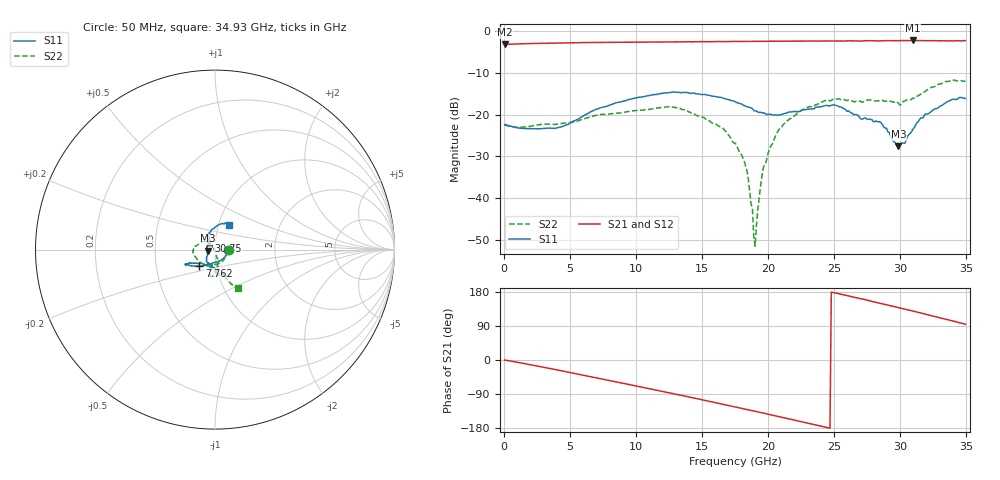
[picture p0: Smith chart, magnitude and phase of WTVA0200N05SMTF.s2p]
! 50 ohm 2-Port S-parameters measured by Modelithics Inc support@modelithics.com  Tampa, FL USA 813-866-6335 (February 2024)
! Smiths Interconnect,  2dB P/N: WTVA0200N05SMTF, Temperature: -50 C
! Board: 10 mil Rogers 4350B, Mounting Pad Dimensions: Length: 15 mils, Width: 25 mils, Gap: 40 mils.
# Hz S RI R 50
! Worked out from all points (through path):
!   352 points, 50 MHz to 34.93 GHz, reference 50 ohm
!   highest |S21| = -2.32 dB at 30.95 GHz (marker M1); lowest = -3.3 dB at 50 MHz (marker M2)
!   group delay of S21, straight-line fit = 21.1 ps
!   lowest |S11| = -27.6 dB at 29.85 GHz (marker M3), VSWR 1.09, Z = 46 - j0.582 ohm
!   |S11| at or under -10 dB: start of sweep to end of sweep
!   |S22| runs from -51.4 to -11.8 dB; largest |S21 - S12| = 0.0048
!   S11 on the Smith chart (normalised r, x): 50 MHz: 1.16, -0.01; 7.762 GHz: 0.83, -0.15; 30.75 GHz: 0.93, +0.09; 34.93 GHz: 1.12, +0.31
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5e7  0.0752 -0.00255  0.686 -0.00206  0.6856 -0.00233  0.0757 -0.00234
3.8815e9  0.0104 -0.0676  0.6451 -0.3032  0.6446 -0.3035  0.0314 -0.0696
5.8715e9  -0.0415 -0.0838  0.56 -0.4554  0.5597 -0.4554  -0.0087 -0.0868
7.762e9  -0.0866 -0.091  0.4415 -0.577  0.4415 -0.5768  -0.048 -0.0888
1.1742e10  -0.1548 -0.0845  0.1121 -0.7237  0.1112 -0.7237  -0.1169 -0.0284
1.5125e10  -0.1527 -0.0825  -0.204 -0.7122  -0.2045 -0.7118  -0.0843 0.0375
1.7513e10  -0.1206 -0.0752  -0.4166 -0.6183  -0.417 -0.6179  -0.0303 0.0338
1.84085e10  -0.0963 -0.0775  -0.4869 -0.5642  -0.4867 -0.5643  -0.0127 0.0166
1.88065e10  -0.0893 -0.0761  -0.518 -0.5392  -0.518 -0.539  -0.00635 0.00426
1.8906e10  -0.0841 -0.0734  -0.5249 -0.5309  -0.525 -0.5306  -0.00213 0.00285
1.90055e10  -0.0803 -0.076  -0.5318 -0.5254  -0.5321 -0.525  -0.000978 -0.00251
1.92045e10  -0.0761 -0.0756  -0.5463 -0.5114  -0.5466 -0.511  0.00117 -0.0071
1.96025e10  -0.067 -0.0802  -0.5735 -0.4829  -0.5732 -0.483  0.00374 -0.0219
2.01995e10  -0.0516 -0.0864  -0.6132 -0.4339  -0.6129 -0.4339  0.00804 -0.0418
2.13935e10  -0.0222 -0.1015  -0.6738 -0.3304  -0.6739 -0.3298  0.0163 -0.082
2.33835e10  -0.000982 -0.1172  -0.7406 -0.1383  -0.7405 -0.1379  0.000789 -0.1228
2.51745e10  0.0049 -0.1286  -0.7522 0.0484  -0.752 0.0487  -0.0199 -0.1524
2.91545e10  -0.0462 -0.0402  -0.6157 0.4482  -0.615 0.4487  0.011 -0.1453
2.9851e10  -0.0413 -0.00631  -0.5684 0.5061  -0.5679 0.5063  0.0231 -0.1349
3.07465e10  -0.0341 0.0487  -0.4988 0.5757  -0.4984 0.5759  0.0483 -0.1422
3.09455e10  -0.0364 0.0557  -0.4845 0.5925  -0.4833 0.5933  0.053 -0.1485
3.49255e10  0.0764 0.1355  -0.0604 0.7594  -0.0572 0.7595  0.1302 -0.2157
